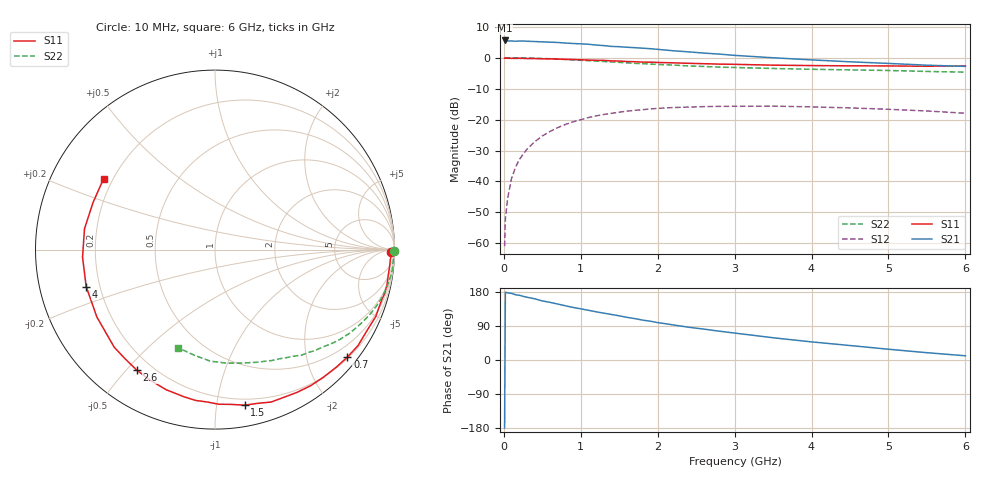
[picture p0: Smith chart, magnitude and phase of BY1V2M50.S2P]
! SIEMENS Small Signal Semiconductors
! BFY420
! Si NPN RF SIEGET Grounded Emitter Transistor in MICRO-X
! VCE = 1.25 V  IC = 0.5 mA
! Common Emitter S-Parameters:  October  1996
# GHz  S  MA  R  50
!  f  S11  S21  S12  S22
! GHz  MAG  ANG  MAG  ANG  MAG  ANG  MAG  ANG
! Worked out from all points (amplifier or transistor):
!   36 points, 10 MHz to 6 GHz, reference 50 ohm
!   highest |S21| = 5.6 dB at 10 MHz (marker M1)
!   |S21| within 3 dB of that: start of sweep to 2.055 GHz
!   unconditionally stable (mu >= 1): 4.727 GHz to end of sweep
!   at 250 MHz: K = 0.03, MSG = 18.3 dB, |S12| = -31.2 dB
!   at 1.4 GHz: K = 0.21, MSG = 10.8 dB, |S12| = -18.0 dB
!   at 6 GHz: K = 1.40, MAG = 3.8 dB, |S12| = -18.0 dB
!   S11 on the Smith chart (normalised r, x): 10 MHz: 71, -40; 700 MHz: 0.23, -2.80; 1.5 GHz: 0.15, -1.20; 2.6 GHz: 0.14, -0.54; 4 GHz: 0.15, -0.14; 6 GHz: 0.16, +0.28
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0.01  0.9789 -0.7  1.901 -179.3  0.0009 97.0  0.9999 -0.3
0.02  0.9837 -1.2  1.896 178.8  0.0025 92.9  0.9972 -0.6
0.05  0.9792 -2.9  1.863 177.2  0.0054 89.2  0.9978 -1.4
0.1  0.9773 -5.7  1.865 175.8  0.0112 88.1  0.9956 -3.0
0.15  0.9756 -8.6  1.847 172.3  0.0167 83.8  0.9943 -4.4
0.2  0.9781 -11.3  1.859 170.8  0.0225 83.0  0.9954 -5.8
0.25  0.9765 -14.3  1.864 168.1  0.0274 80.7  0.9923 -7.3
0.4  0.9703 -22.6  1.827 161.6  0.0437 75.6  0.9821 -11.5
0.5  0.9593 -28.3  1.805 155.9  0.0543 71.8  0.9725 -14.4
0.7  0.9504 -39.1  1.764 147.7  0.0742 64.9  0.9507 -19.7
0.9  0.933 -49.8  1.697 138.7  0.092 57.8  0.9238 -24.7
1.1  0.9172 -60.2  1.65 131.2  0.1079 51.2  0.8962 -29.5
1.5  0.8823 -79.2  1.507 116.6  0.1318 39.1  0.8408 -38.0
1.8  0.8502 -92.9  1.427 105.4  0.1444 31.4  0.801 -43.5
2.2  0.8269 -109.2  1.296 92.7  0.1566 21.7  0.7612 -50.5
2.6  0.8007 -122.9  1.189 81.5  0.162 13.9  0.7215 -56.6
3  0.7818 -135.9  1.091 71.1  0.164 6.8  0.6949 -62.7
3.5  0.7578 -150.3  0.998 58.7  0.1651 -0.5  0.6704 -69.4
4  0.7466 -164.0  0.922 47.8  0.1605 -7.1  0.6498 -76.6
4.5  0.7392 -176.7  0.859 38.2  0.1545 -12.7  0.6361 -84.1
5.5  0.7284 158.9  0.757 19.3  0.1377 -20.5  0.5997 -101.1
6  0.7358 147.5  0.724 11.1  0.1266 -22.0  0.5842 -110.7
